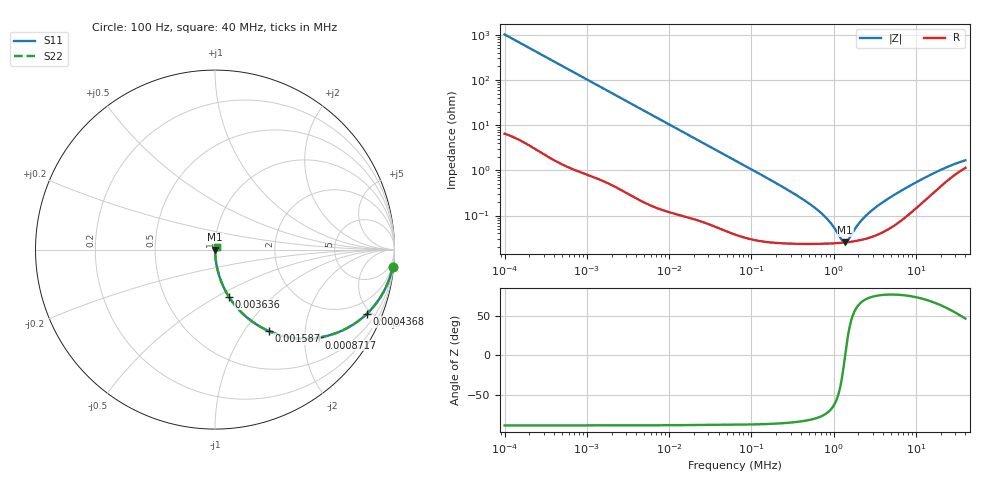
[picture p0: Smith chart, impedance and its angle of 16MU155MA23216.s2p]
!Components F PML CAP
!CONCATENATE F 0.1-40000kHz, at 20deg DC=0V
!Part Number F 16MU155MA23216
!Copyright(C) Rubycon Corporation. 20161128
# MHz S MA R 50
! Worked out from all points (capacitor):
!   561 points, 100 Hz to 40 MHz, reference 50 ohm
!   read as one part in series: C = 1.56 uF near 104.7 Hz
!   lowest |Z| = 25.4 mohm at 1.385 MHz (marker M1)
!   series resonance near 1.38 MHz, so ESL is about 8.5 nH
!   S11 on the Smith chart (normalised r, x): 100 Hz: 1, -20; 436.8 Hz: 1.03, -4.69; 871.7 Hz: 1.02, -2.36; 1.587 kHz: 1.01, -1.30; 3.636 kHz: 1.01, -0.57; 40 MHz: 1.02, +0.02
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0.0001  0.9946 -5.6  0.09774 84.0  0.09774 84.0  0.9946 -5.6
0.0002399605  0.9721 -13.2  0.2281 76.4  0.2281 76.4  0.9721 -13.2
0.0004367525  0.9178 -23.0  0.3911 66.6  0.3911 66.6  0.9178 -23.0
0.0008716573  0.7597 -40.1  0.6446 49.4  0.6446 49.4  0.7597 -40.1
0.001586505  0.5426 -56.6  0.8352 32.9  0.8352 32.9  0.5426 -56.6
0.002346951  0.4016 -65.8  0.9121 23.7  0.9121 23.7  0.4016 -65.8
0.003635581  0.2734 -73.6  0.9594 15.9  0.9594 15.9  0.2734 -73.6
0.007424854  0.1384 -81.5  0.989 8.0  0.989 8.0  0.1384 -81.5
0.01823188  0.05715 -85.9  0.9975 3.3  0.9975 3.3  0.05715 -85.9
0.06324555  0.01668 -87.7  0.9995 1.0  0.9995 1.0  0.01668 -87.7
0.2637898  0.003883 -86.2  0.9998 0.2  0.9998 0.2  0.003883 -86.2
0.5512845  0.001635 -81.6  0.9998 0.1  0.9998 0.1  0.001635 -81.6
0.8345301  0.0008412 -73.5  0.9998 0.0  0.9998 0.0  0.0008412 -73.5
1.003394  0.0005543 -64.1  0.9998 0.0  0.9998 0.0  0.0005543 -64.1
1.263305  0.0002842 -28.6  0.9998 0.0  0.9998 0.0  0.0002842 -28.6
1.385233  0.0002535 1.3  0.9997 -0.0  0.9997 -0.0  0.0002535 1.3
1.484342  0.0002802 23.5  0.9997 -0.0  0.9997 -0.0  0.0002802 23.5
1.912381  0.0005791 61.6  0.9997 -0.0  0.9997 -0.0  0.0005791 61.6
2.407749  0.0009475 71.4  0.9997 -0.1  0.9997 -0.1  0.0009475 71.4
4.69589  0.002417 77.8  0.9995 -0.1  0.9995 -0.1  0.002417 77.8
15.91889  0.00835 68.2  0.9969 -0.4  0.9969 -0.4  0.00835 68.2
40  0.01651 46.6  0.9887 -0.7  0.9887 -0.7  0.01651 46.6
